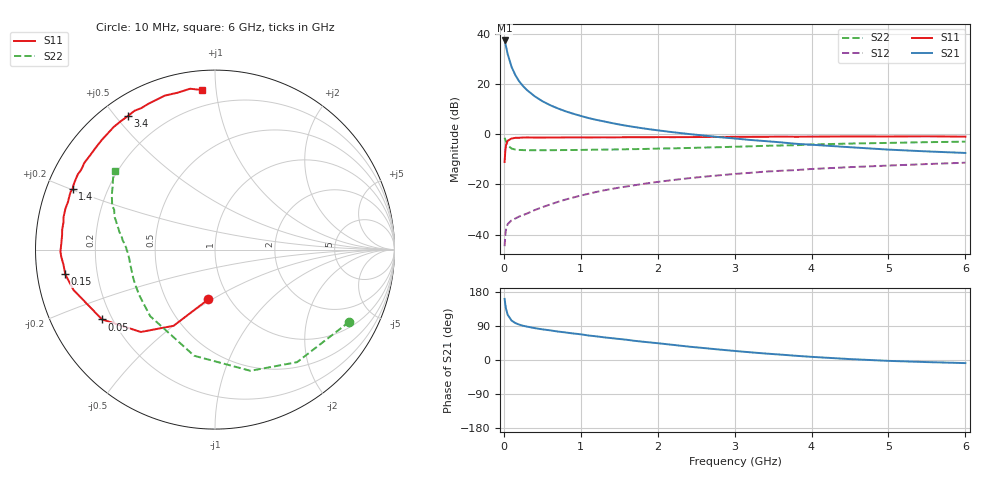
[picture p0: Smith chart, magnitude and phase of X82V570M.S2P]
! SIEMENS Small Signal Semiconductors
! BFP136W
! Si NPN RF Bipolar Junction Transistor in SOT343
! VCE = 2.5 V  IC = 70 mA
! Common Emitter S-Parameters:  September  1994
# GHz  S  MA  R  50
!  f  S11  S21  S12  S22
! GHz  MAG  ANG  MAG  ANG  MAG  ANG  MAG  ANG
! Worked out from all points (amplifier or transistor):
!   40 points, 10 MHz to 6 GHz, reference 50 ohm
!   highest |S21| = 37.3 dB at 10 MHz (marker M1)
!   |S21| within 3 dB of that: start of sweep to 32.81 MHz
!   unconditionally stable (mu >= 1): 519.2 MHz to 2.879 GHz
!   at 200 MHz: K = 0.63, MSG = 26.9 dB, |S12| = -32.8 dB
!   at 1.5 GHz: K = 1.10, MAG = 10.6 dB, |S12| = -21.3 dB
!   at 6 GHz: K = 0.96, MSG = 1.9 dB, |S12| = -11.4 dB
!   S11 on the Smith chart (normalised r, x): 10 MHz: 0.80, -0.48; 50 MHz: 0.16, -0.28; 150 MHz: 0.08, -0.08; 1.4 GHz: 0.08, +0.20; 3.4 GHz: 0.08, +0.54; 6 GHz: 0.11, +0.92
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0.01  0.2798 -97.7  73.36 161.2  0.0059 71.2  0.8499 -28.2
0.02  0.483 -118.5  63.75 145.3  0.0101 57.4  0.7762 -53.9
0.03  0.6177 -132.0  54.36 133.7  0.0132 50.2  0.7036 -73.7
0.05  0.74 -148.3  39.29 119.3  0.0162 39.0  0.6027 -101.1
0.1  0.82 -164.1  21.91 104.2  0.0193 33.7  0.5177 -134.2
0.15  0.8455 -170.6  14.93 97.4  0.021 36.1  0.4931 -148.4
0.2  0.8484 -174.3  11.22 93.4  0.023 38.6  0.4856 -156.1
0.25  0.857 -177.2  9.05 90.3  0.0245 41.3  0.4823 -161.0
0.3  0.8613 -179.2  7.568 88.2  0.0263 44.1  0.4794 -164.3
0.4  0.8566 177.2  5.698 84.2  0.0308 49.7  0.4791 -168.6
0.5  0.8558 174.4  4.54 80.9  0.0352 52.5  0.4795 -171.5
0.6  0.8588 172.5  3.791 78.3  0.0398 55.6  0.48 -173.4
0.7  0.8577 169.8  3.266 75.2  0.0448 57.7  0.4815 -174.7
0.9  0.8633 166.3  2.557 70.1  0.0547 59.1  0.4841 -177.3
1.1  0.8612 162.0  2.093 64.6  0.0651 60.2  0.4887 -178.8
1.4  0.8628 156.9  1.669 57.7  0.0812 60.2  0.4947 178.8
2.2  0.8718 143.0  1.093 39.9  0.1224 55.4  0.5217 172.9
3.2  0.8873 126.2  0.768 20.4  0.1701 46.2  0.5726 164.1
3.4  0.8883 123.2  0.728 17.1  0.1799 44.1  0.5866 162.2
4.5  0.9024 108.1  0.55 2.4  0.2207 33.9  0.6506 152.1
5.5  0.907 98.8  0.454 -5.5  0.2542 25.9  0.6933 145.0
6  0.8917 94.5  0.423 -8.2  0.2705 21.5  0.709 141.9
